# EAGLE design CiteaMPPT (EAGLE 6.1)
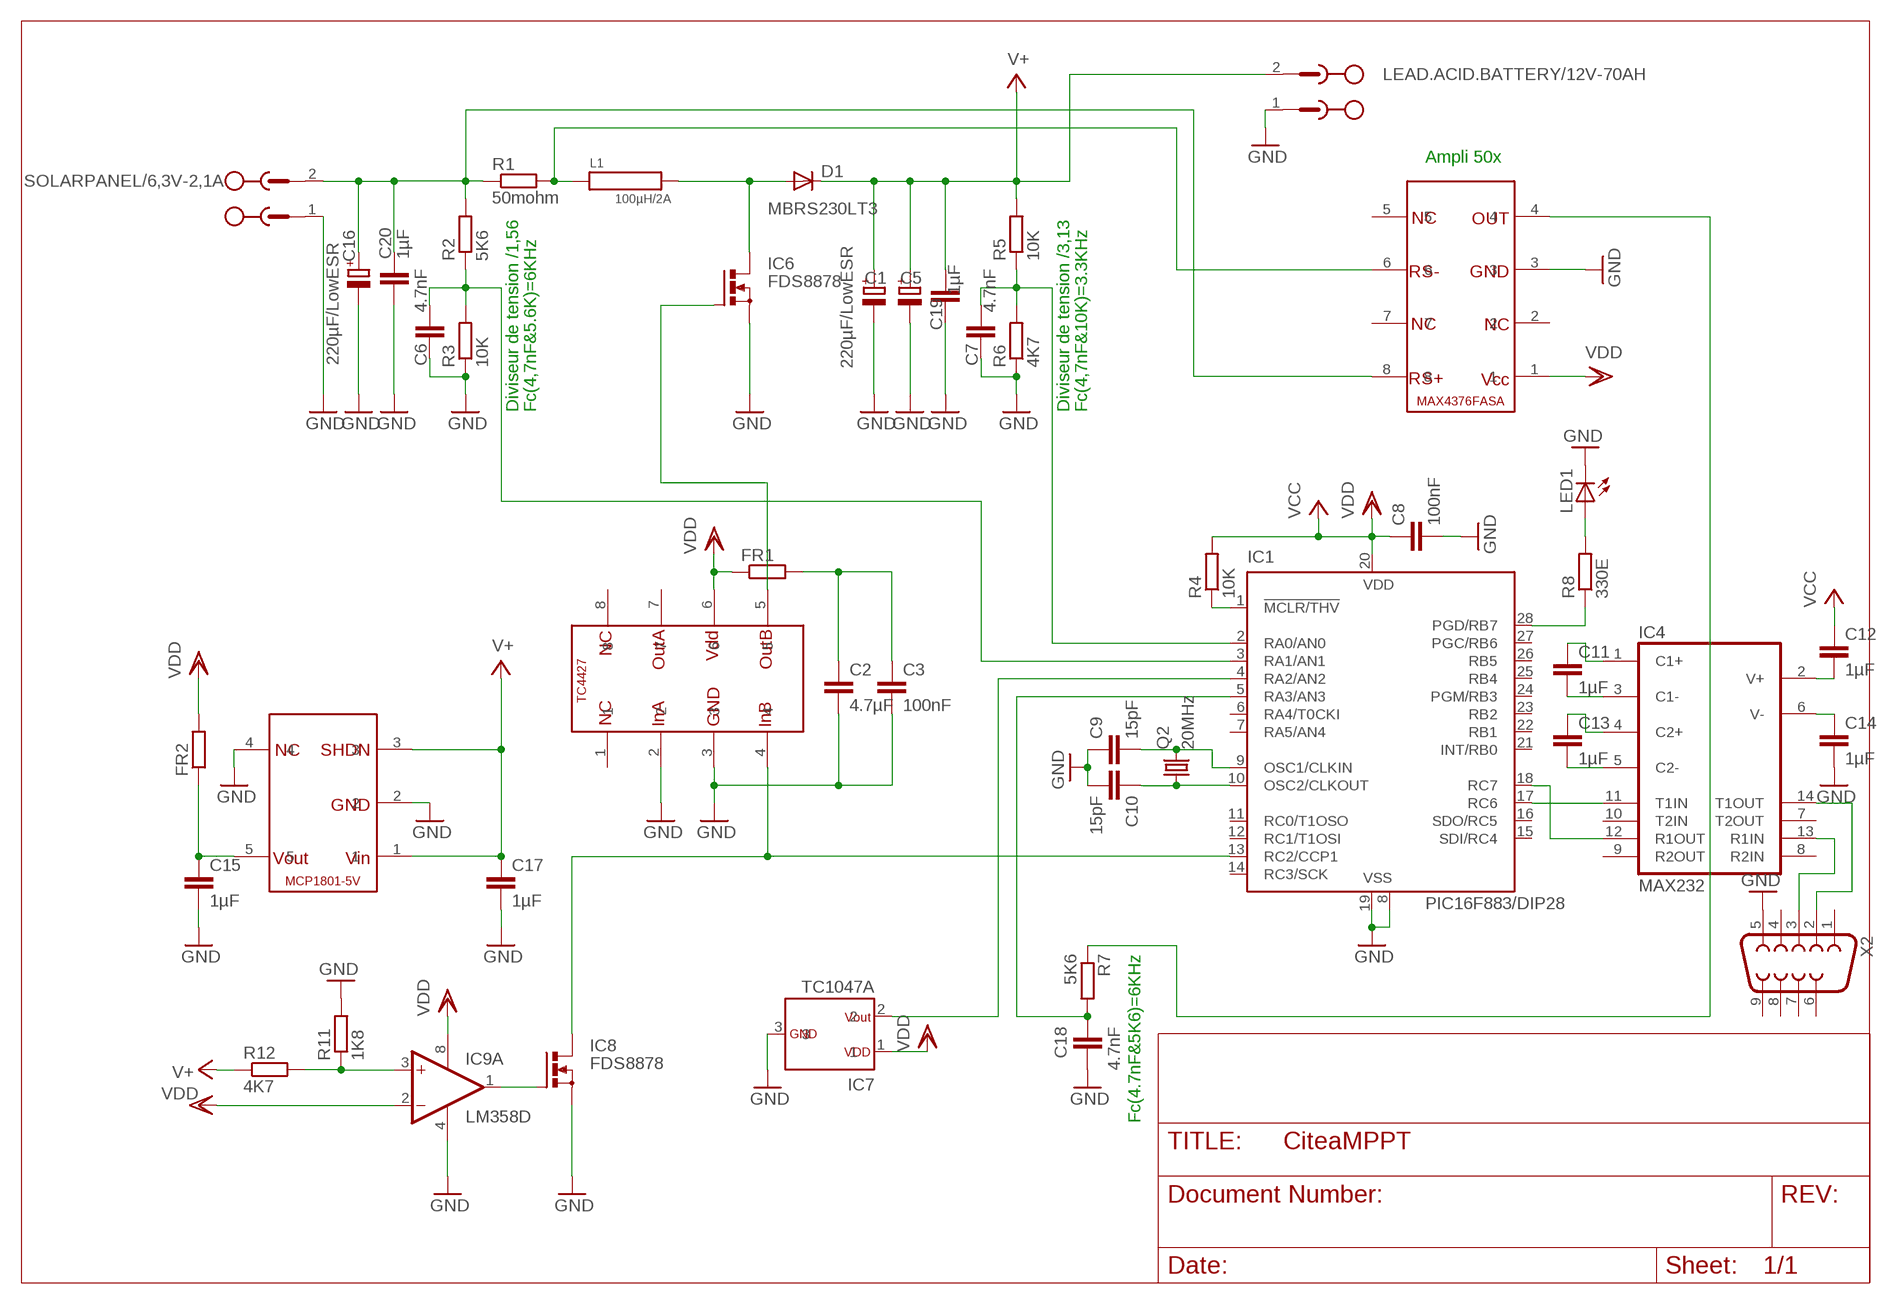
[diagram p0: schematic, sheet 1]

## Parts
C1  220µF/LowESR  CPOL-EUE3.5-8  [E3,5-8]
C2  4.7µF  C-EUC0805  [C0805]
C3  100nF  C-EUC0805  [C0805]
C5  220µF/LowESR  CPOL-EUE3.5-8  [E3,5-8]
C6  4.7nF  C-EUC0805  [C0805]
C7  4.7nF  C-EUC0805  [C0805]
C8  100nF  C-EUC0805  [C0805]
C9  15pF  C-EUC0805  [C0805]
C10  15pF  C-EUC0805  [C0805]
C11  1µF  C-EUC0805  [C0805]
C12  1µF  C-EUC0805  [C0805]
C13  1µF  C-EUC0805  [C0805]
C14  1µF  C-EUC0805  [C0805]
C15  1µF  C-EUC0805  [C0805]
C16  220µF/LowESR  CPOL-EUE3.5-8  [E3,5-8]
C17  1µF  C-EUC0805  [C0805]
C18  4.7nF  C-EUC0805  [C0805]
C19  1µF  C-EUC0805  [C0805]
C20  1µF  C-EUC0805  [C0805]
D1  MBRS230LT3  DIODE-SMB  [SMB]
FR1  R-EU_M0805  [M0805]
FR2  R-EU_M0805  [M0805]
IC1  PIC16F883/DIP28  PIC16F872P  [DIL28-3]
IC2  MAX4376  [MAX4376]
IC3  TC4427  [TC4427]
IC4  MAX232  [DIL16]
IC5  MCP1801-5V  [MCP1801-5V]
IC6  FDS8878  [FDS8878]
IC7  TC1047A  [TC1047A]
IC8  FDS8878  [FDS8878]
IC9  LM358D  [SO08]
L1  100µH/2A  WE/INDUCTOR/SMD/.100  [WE.100]
LEAD.ACID.BATTERY/12V-70AH  CONPHENIX  [CONPHENIX]
LED1  LEDCHIPLED_1206  [CHIPLED_1206]
Q2  20MHz  CRYSTALHC49S  [HC49/S]
R1  50mohm  R-EU_R1206  [R1206]
R2  5K6  R-EU_M0805  [M0805]
R3  10K  R-EU_M0805  [M0805]
R4  10K  R-EU_M0805  [M0805]
R5  10K  R-EU_M0805  [M0805]
R6  4K7  R-EU_M0805  [M0805]
R7  5K6  R-EU_M0805  [M0805]
R8  330E  R-EU_M0805  [M0805]
R11  1K8  R-EU_M0805  [M0805]
R12  4K7  R-EU_M0805  [M0805]
SOLARPANEL/6,3V-2,1A  CONPHENIX  [CONPHENIX]
X2  F09VP  [F09VP]

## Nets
GND: C1.- C2.2 C3.2 C5.- C6.2 C7.2 C8.2 C9.1 C10.2 C14.2 C15.2 C16.- C17.2 C18.1 C19.2 C20.2 IC1.8(VSS) IC1.19(VSS) IC2.3 IC3.2 IC3.3 IC5.2 IC5.4 IC6.1 IC6.2 IC6.3 IC7.3 IC8.1 IC8.2 IC8.3 IC9.4(P:V-) LEAD.ACID.BATTERY/12V-70AH.1 LED1.C R3.1 R6.1 R11.2 SOLARPANEL/6,3V-2,1A.1 X2.5
N$1: C6.1 IC1.3(RA1/AN1) R2.1 R3.2
N$2: IC2.6 L1.2 R1.2
N$3: C16.+ C20.1 IC2.8 R1.1 R2.2 SOLARPANEL/6,3V-2,1A.2
N$4: D1.A IC6.5 IC6.6 IC6.7 IC6.8 L1.1
N$5: IC8.4 IC9.1(A:OUT)
N$6: LED1.A R8.2
N$7: C9.2 IC1.9(OSC1/CLKIN) Q2.2
N$8: C18.2 IC1.5(RA3/AN3) R7.2
N$9: C7.1 IC1.2(RA0/AN0) R5.1 R6.2
N$10: IC1.13(RC2/CCP1) IC3.4 IC8.5 IC8.6 IC8.7 IC8.8
N$11: IC1.4(RA2/AN2) IC7.2
N$12: IC1.28(PGD/RB7) R8.1
N$13: IC2.4 R7.1
N$14: C10.1 IC1.10(OSC2/CLKOUT) Q2.1
N$15: C11.2 IC4.3(C1-)
N$16: C11.1 IC4.1(C1+)
N$17: C13.1 IC4.4(C2+)
N$18: C13.2 IC4.5(C2-)
N$19: C12.2 IC4.2(V+)
N$20: C14.1 IC4.6(V-)
N$21: IC1.18(RC7) IC4.12(R1OUT)
N$22: IC1.17(RC6) IC4.11(T1IN)
N$23: IC4.13(R1IN) X2.3
N$24: IC4.14(T1OUT) X2.2
N$25: C2.1 C3.1 FR1.2
N$26: IC3.5 IC6.4
N$27: IC1.1(!MCLR/THV) R4.1
N$28: C15.1 FR2.1 IC5.5
N$29: IC9.3(A:+IN) R11.1 R12.2
V+: C1.+ C5.+ C17.1 C19.1 D1.C IC5.1 IC5.3 LEAD.ACID.BATTERY/12V-70AH.2 R5.2 R12.1
VCC: C8.1 C12.1 IC1.20(VDD) R4.2 ; supply symbol labelled VDD
VDD: FR1.1 FR2.2 IC2.1 IC3.6 IC7.1 IC9.2(A:-IN) IC9.8(P:V+)
Unconnected: IC1.6(RA4/T0CKI) IC1.7(RA5/AN4) IC1.11(RC0/T1OSO) IC1.12(RC1/T1OSI) IC1.14(RC3/SCK) IC1.15(SDI/RC4) IC1.16(SDO/RC5) IC1.21(INT/RB0) IC1.22(RB1) IC1.23(RB2) IC1.24(PGM/RB3) IC1.25(RB4) IC1.26(RB5) IC1.27(PGC/RB6) IC2.2 IC2.5 IC2.7 IC3.1 IC3.7 IC3.8 IC4.7(T2OUT) IC4.8(R2IN) IC4.9(R2OUT) IC4.10(T2IN) IC9.5(B:+IN) IC9.6(B:-IN) IC9.7(B:OUT) X2.1 X2.4 X2.6 X2.7 X2.8 X2.9

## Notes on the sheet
- Ampli 50x
- Diviseur de tension /1,56 | Fc(4,7nF&5.6K)=6KHz | Diviseur de tension /3,13 | Fc(4,7nF&10K)=3.3KHz
- Fc(4.7nF&5K6)=6KHz

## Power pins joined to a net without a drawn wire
GND: IC4.15(GND)
VCC: IC4.16(VCC)

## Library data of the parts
C1 C5 C16 = rcl:CPOL-EU: POLARIZED CAPACITOR, European symbol
C2 C3 C6-C15 C17-C20 = rcl:C-EU: CAPACITOR, European symbol
D1 = diode:DIODE-: DIODE
FR1 FR2 R1-R8 R11 R12 = rcl:R-EU_: RESISTOR, European symbol
IC1 = microchip:PIC16*872: MICROCONTROLLER flash type; MF: MICROCHIP; MPN: PIC16F872-I/SP; OC_FARNELL: 9761012; OC_NEWARK: 12C1945
IC2 = solarRegulator:MAX4376
IC3 = solarRegulator:TC4427
IC4 = maxim:MAX232: RS232 TRANSEIVER; MF: MAXIM; MPN: MAX232ACPE+; OC_FARNELL: 9723773; OC_NEWARK: 68K4544
IC5 = solarRegulator:MCP1801-5V
IC6 IC8 = solarRegulator:FDS8878
IC7 = solarRegulator:TC1047A
IC9 = linear:LM358: OP AMP also LM158; LM258; LM2904 Source: http://cache.national.com/ds/LM/LM158.pdf
L1 = solarRegulator:WE/INDUCTOR/SMD/.100
LEAD.ACID.BATTERY/12V-70AH SOLARPANEL/6,3V-2,1A = solarRegulator:CONPHENIX
LED1 = led:LED: LED
Q2 = crystal:CRYSTAL: CRYSTAL; OC_FARNELL: 1667008; OC_NEWARK: unknown
X2 = con-subd:F09: SUB-D; OC_FARNELL: unknown; OC_NEWARK: unknown

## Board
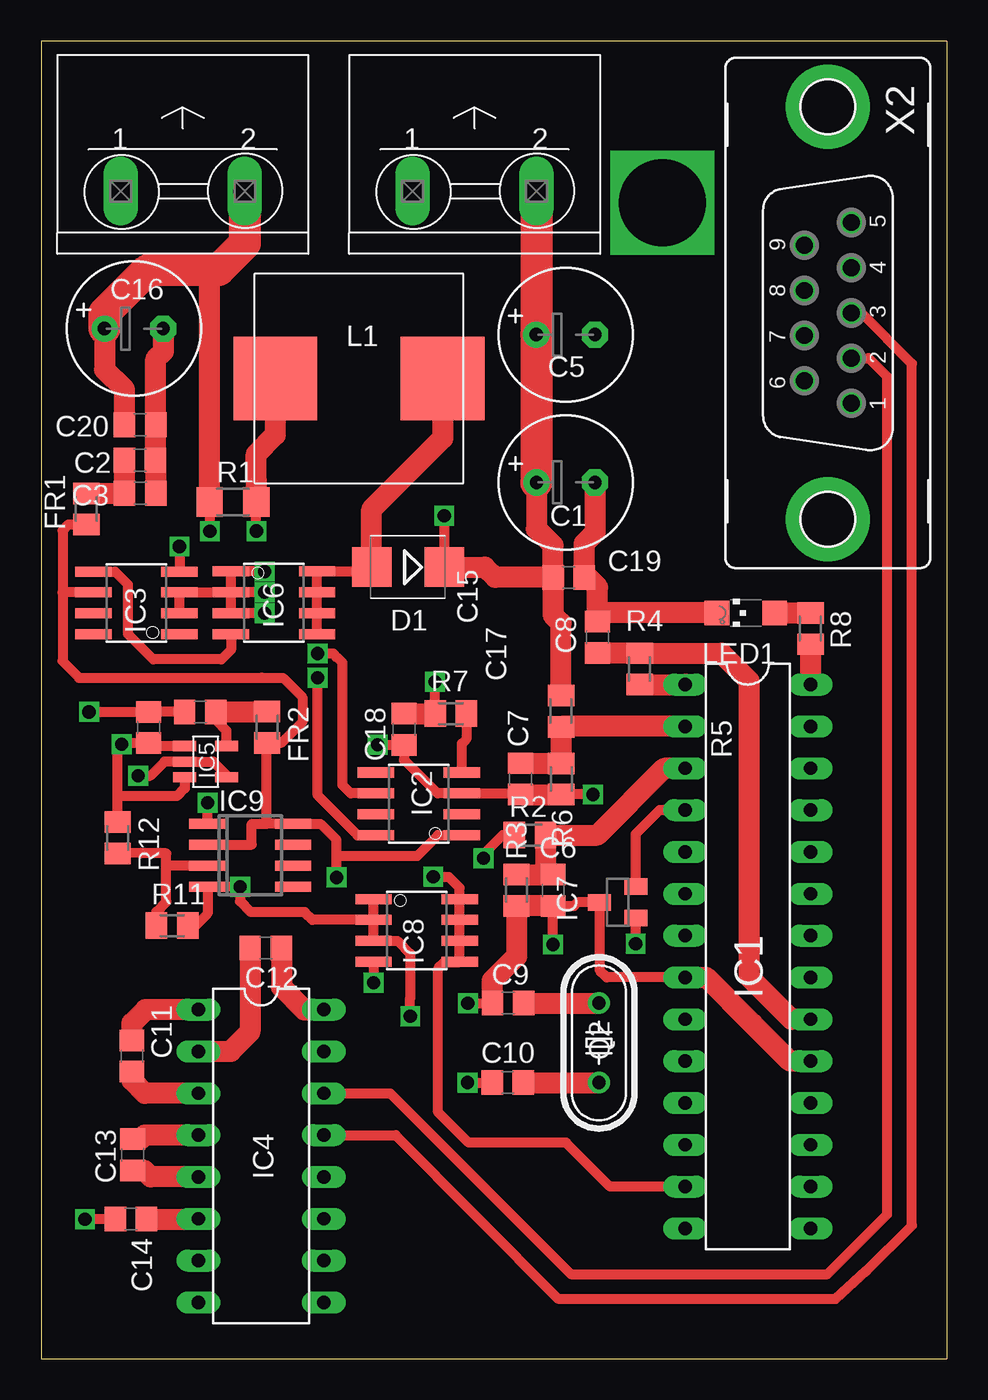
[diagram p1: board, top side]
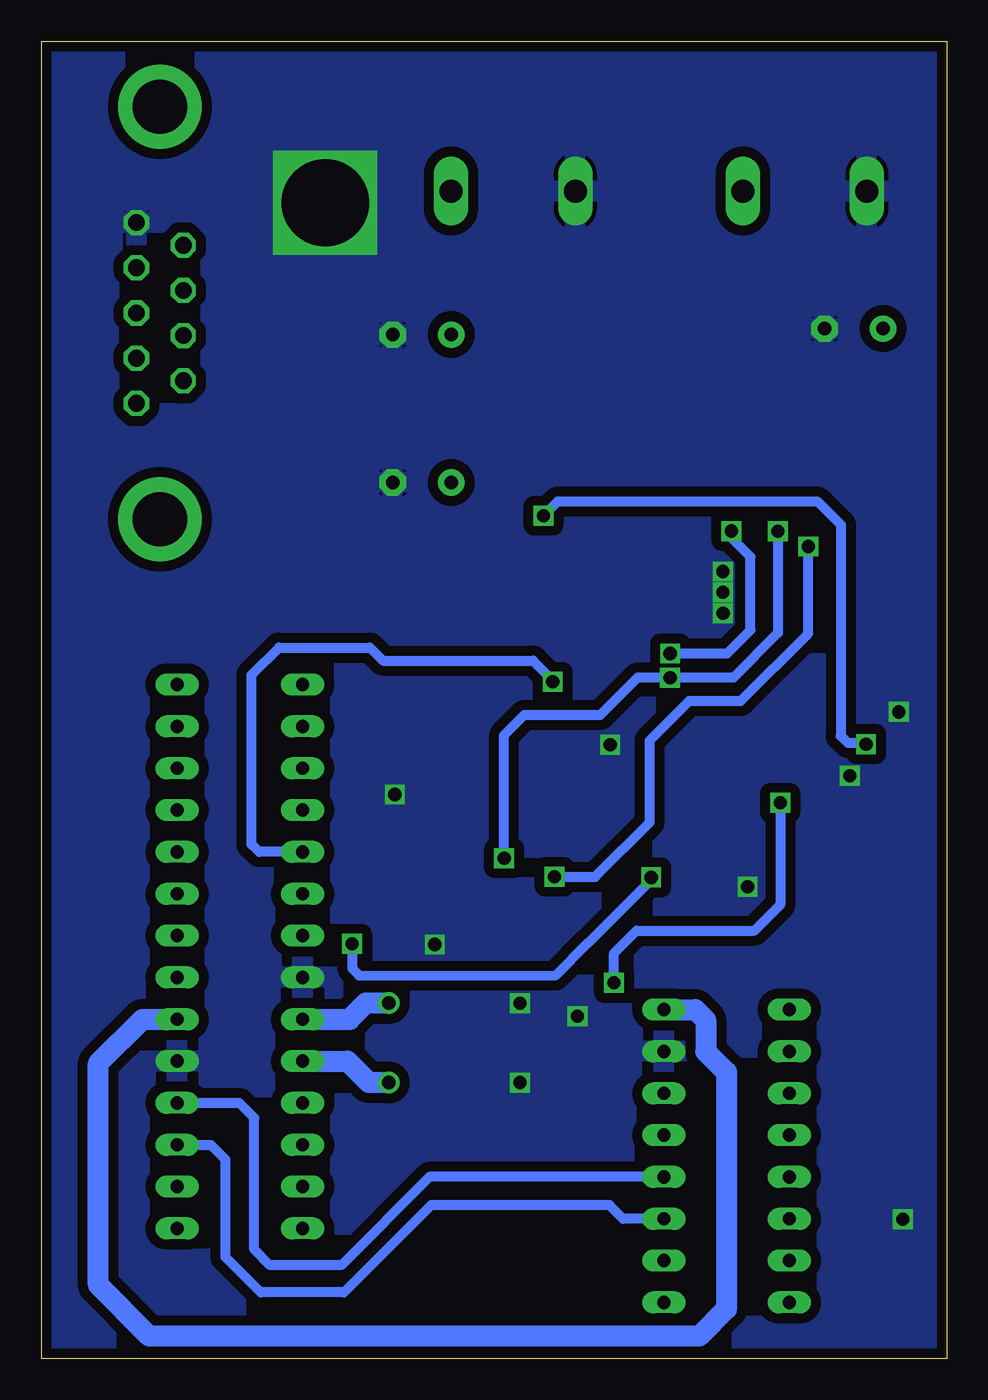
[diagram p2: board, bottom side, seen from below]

Size 55 x 80 mm. Coordinates in mm from the lower left corner, seen from the top.
Outline: 0,0 55,0 55,80 0,80 0,0
Copper layers (1*16): Top 0.035mm / dielectric 1.5mm / Bottom 0.035mm
Design rules: minimum track width 10mil, minimum drill 24mil, track to track 8mil, track to pad 8mil, pad to pad 8mil, via to via 8mil, smd to smd 8mil, copper to edge 10mil, drill to drill 8mil, minimum pad ring 10mil, minimum via ring 8mil, stop-mask expansion 4mil, vias tented up to drill 0mil, thermal gap 10mil

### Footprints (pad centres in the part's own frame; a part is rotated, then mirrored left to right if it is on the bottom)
E3,5-8 = drill 0.813 pad 1.6: + -1.778,0 | drill 0.813 pad 1.6 octagon: - 1.778,0
C0805 = smd 1.3 x 1.5: 1 -0.95,0; 2 0.95,0
SMB = smd 2.4 x 2.4: A 2.2,0; C -2.2,0
M0805 = smd 1.3 x 1.6: 1 -0.95,0; 2 0.95,0
DIL28-3 = drill 0.813 long: 1 -16.51,-3.81; 2 -13.97,-3.81; 3 -11.43,-3.81; 4 -8.89,-3.81; 5 -6.35,-3.81; 6 -3.81,-3.81; 7 -1.27,-3.81; 8 1.27,-3.81; 9 3.81,-3.81; 10 6.35,-3.81; 11 8.89,-3.81; 12 11.43,-3.81; 13 13.97,-3.81; 14 16.51,-3.81; 15 16.51,3.81; 16 13.97,3.81; 17 11.43,3.81; 18 8.89,3.81; 19 6.35,3.81; 20 3.81,3.81; 21 1.27,3.81; 22 -1.27,3.81; 23 -3.81,3.81; 24 -6.35,3.81; 25 -8.89,3.81; 26 -11.43,3.81; 27 -13.97,3.81; 28 -16.51,3.81
MAX4376 = smd 2.21 x 0.61: 1 -2.616,1.905; 2 -2.616,0.635; 3 -2.616,-0.635; 4 -2.616,-1.905; 5 2.616,-1.905; 6 2.616,-0.635; 7 2.616,0.635; 8 2.616,1.905
TC4427 = smd 2.21 x 0.61: 1 -2.616,1.905; 2 -2.616,0.635; 3 -2.616,-0.635; 4 -2.616,-1.905; 5 2.616,-1.905; 6 2.616,-0.635; 7 2.616,0.635; 8 2.616,1.905
DIL16 = drill 0.813 long: 1 -8.89,-3.81; 2 -6.35,-3.81; 3 -3.81,-3.81; 4 -1.27,-3.81; 5 1.27,-3.81; 6 3.81,-3.81; 7 6.35,-3.81; 8 8.89,-3.81; 9 8.89,3.81; 10 6.35,3.81; 11 3.81,3.81; 12 1.27,3.81; 13 -1.27,3.81; 14 -3.81,3.81; 15 -6.35,3.81; 16 -8.89,3.81
MCP1801-5V = smd 0.61 x 1.397: 1 -0.953,-1.27; 2 0,-1.27; 3 0.953,-1.27; 4 0.953,1.27; 5 -0.953,1.27
FDS8878 = smd 2.21 x 0.61: 1 -2.616,1.905; 2 -2.616,0.635; 3 -2.616,-0.635; 4 -2.616,-1.905; 5 2.616,-1.905; 6 2.616,-0.635; 7 2.616,0.635; 8 2.616,1.905
TC1047A = smd 1 x 1.4: 1 -0.95,-1.1; 2 0.95,-1.1; 3 0,1.1
SO08 = smd 0.6 x 2.2: 1 -1.905,-2.6; 2 -0.635,-2.6; 3 0.635,-2.6; 4 1.905,-2.6; 5 1.905,2.6; 6 0.635,2.6; 7 -0.635,2.6; 8 -1.905,2.6
WE.100 = smd 5.08 x 5.08: 1 -5.08,0; 2 5.08,0
CONPHENIX = drill 1.397 long: 1 4.405,0; 2 -3.135,0
CHIPLED_1206 = smd 1.5 x 1.5: A 0,-1.75; C 0,1.75
HC49/S = drill 0.813: 1 -2.413,0; 2 2.413,0
R1206 = smd 1.6 x 1.803: 1 -1.422,0; 2 1.422,0
F09VP = drill 1.016 octagon: 1 5.486,1.422; 2 2.743,1.422; 3 0,1.422; 4 -2.743,1.422; 5 -5.486,1.422; 6 4.115,-1.422; 7 1.372,-1.422; 8 -1.372,-1.422; 9 -4.115,-1.422 | drill 3.302 pad 5.08: G1 -12.522,0; G2 12.522,0

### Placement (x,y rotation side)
C1  31.87,53.21 0 top
C2  6,54.56 0 top
C3  6.02,52.55 0 top
C5  31.86,62.18 0 top
C6  31.11,28.45 270 top
C7  29.11,35.21 270 top
C8  33.79,43.81 90 top
C9  28.36,21.6 0 top
C10  28.34,16.77 180 top
C11  5.52,18.38 270 top
C12  13.64,24.94 180 top
C13  5.56,12.39 270 top
C14  5.46,8.48 180 top
C15  9.67,39.28 180 top
C16  5.63,62.54 0 top
C17  6.54,38.33 90 top
C18  22.04,38.22 90 top
C19  32.05,47.44 0 top
C20  6.01,56.71 0 top
D1  22.27,48.07 180 top
FR1  2.75,51.6 90 top
FR2  13.73,38.34 270 top
IC1  42.93,24.43 270 top
IC2  22.94,33.69 180 top
IC3  5.78,45.89 180 top
IC4  13.36,12.31 270 top
IC5  9.99,36.25 270 top
IC6  14.14,45.9 0 top
IC7  35.02,27.72 90 top
IC8  22.81,26.01 0 top
IC9  12.7,30.58 270 top
L1  19.31,59.52 180 top
LEAD.ACID.BATTERY/12V-70AH  26.96,70.9 180 top
LED1  42.8,45.29 90 top
Q2  33.88,19.19 90 top
R1  11.65,52.02 0 top
R2  29.68,31.8 180 top
R3  28.87,28.45 90 top
R4  36.35,41.89 90 top
R5  31.59,39.32 90 top
R6  31.59,35.2 90 top
R7  24.88,39.17 180 top
R8  46.73,44.33 90 top
R11  7.96,26.3 0 top
R12  4.65,31.63 270 top
SOLARPANEL/6,3V-2,1A  9.24,70.9 180 top
X2  47.79,63.5 270 top

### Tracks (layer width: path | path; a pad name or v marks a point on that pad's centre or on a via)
GND  (via drill 0.8, 5.3)
  Top 0.61: IC6.2 IC6.3 11.56,45.26 11.56,45.27 | IC6.2 IC6.1 | IC3.2 IC3.3 IC6.2 | v13.58,46.53 12.42,46.54 12.43,46.53 | 12.43,46.54 12.43,46.53 | IC6.2 12.43,46.53 | v13.58,47.8 IC6.1 | IC6.1 | v13.58,45.27 11.56,45.27 | 11.56,45.27 11.56,45.31 | IC5.4 11.26,35.44 10.45,36.26 IC5.2 7.5,36.26 6.65,35.41 v5.89,35.41 | R11.2 9.37,26.3 10.1,27.03 IC9.4 | C15.2 8.7,39.29 C17.2 | C7.2 29.06,34.31 29.06,34.34 29.05,34.33 IC2.3 24.08,34.33 22.04,36.37 C18.1 v20.43,37.27 | IC9.4 v12.08,28.67 12.08,27.77 12.74,27.12 16.01,27.12 16.48,26.65 IC8.2 | 10.09,28.67 IC9.4 | IC9.4 | 6.53,39.28 | 6.53,39.28 C17.2 | C17.2 | v25.92,21.59 27.39,21.59 27.41,21.59 C9.1 | v25.91,16.77 C10.2 | IC8.2 IC8.3 21.65,25.38 22.42,24.6 22.42,21.9 | IC8.2 20.2,27.79 20.17,27.79 20.17,27.74 | IC8.2 IC8.1 20.19,27.9 20.2,27.9 | IC1.8 34.36,23.16 33.92,23.6 33.92,23.61 IC7.3 32.59,27.72 32.37,27.5 C6.2 31.09,27.48 v31.09,25.15 | v33.52,34.26 31.58,34.26 31.55,34.3 R6.1 | 22.42,21.9 22.41,21.9 | v22.42,20.81 22.42,21.9 22.42,21.91 22.42,21.9 | v2.91,39.28 C17.2 | C17.2 | C14.2 v2.67,8.48 v2.66,8.48
  Top 1.27: C1.- 33.64,50.16 33,49.51 C19.2 33.2,47.44 33.81,46.84 33.79,46.82 C8.2 33.76,44.78 33.76,44.87 34.18,45.29 LED1.C | C16.- 7.41,61.16 6.96,60.7 C20.2 C2.2 6.95,52.56 C3.2 | C15.2 | C7.2 R6.1 | C6.2 R3.1 28.87,24.43 27.41,22.97 C9.1 | IC1.8 40.4,23.16 43.2,20.36 | IC1.19 45.48,18.08 43.2,20.36 | 43.2,20.36 | 43.2,20.36 43.2,20.35
  other vias: 37.74,70.19
  pour Bottom (isolate 0.61): 1,79 54,79 54,1 1,1
N$1
  Top 1.27: R3.2 31.12,29.4 31.14,29.39 C6.1 30.72,29.4 30.63,29.49 R2.1 33.78,31.8 37.84,35.86 IC1.3
N$2  (via drill 0.8)
  Top 0.61: v13.07,50.26 13.07,50.33 R1.2 | IC2.6 18.81,34.33 18.3,34.84 18.3,41.97 | 18.3,41.97 | v16.79,42.82 17.74,42.82 18.02,42.55 | 18.02,42.55 18.03,42.55 | 18.3,41.97 18.3,42.27 18.02,42.55
  Top 1.27: R1.2 13.07,54.94 14.23,56.09 L1.2
  Bottom 0.61: v16.79,42.82 13.32,42.82 11.91,44.24 11.91,48.69 13.07,49.85 v13.07,50.26 13.07,50.33
N$3  (via drill 0.8)
  Top 0.61: v10.25,50.25 10.25,50.35 10.25,52.03 10.25,52.02 R1.1 | IC2.8 19.21,31.79 16.8,34.2 v16.8,41.36 | v26.88,30.39 26.88,30.64 28.03,31.8 R2.2
  Top 1.27: R1.1 10.23,65.72 10.63,66.12 | C20.1 5.06,58.86 3.86,60.06 C16.+
  Top 1.93: C16.+ 3.86,63.5 6.48,66.12 10.63,66.12 10.79,66.12 12.37,67.7 SOLARPANEL/6,3V-2,1A.2
  Bottom 0.61: v10.25,50.25 10.24,44.07 12.95,41.36 16.64,41.36 v16.8,41.36 18.77,41.36 21.03,39.1 25.64,39.1 26.88,37.87 v26.88,30.39
N$4
  Top 0.61: IC6.5 IC6.6 IC6.7 IC6.8 19.81,47.8 20,48 | 20,48 | 20,48 D1.A
  Top 1.27: D1.A 20.07,51.57 24.39,55.88 L1.1
N$5  (via drill 0.8)
  Top 0.61: IC8.4 v20.2,22.83 v20.2,22.82 | IC9.1 v10.1,33.75 v10.11,33.76
  Bottom 0.61: v20.2,22.82 20.2,24.63 18.84,25.99 11.67,25.99 10.11,27.55 v10.11,33.76
N$6
  Top 1.27: LED1.A R8.2
N$7
  Top 1.27: C9.2 Q2.2 33.9,21.61 Q2.2
  Bottom 1.27: Q2.2 35.28,21.6 36.26,20.62 IC1.9
N$8  (via drill 0.8)
  Top 0.61: C18.2 | R7.2 v23.93,41.1
  Top 1.27: C18.2 R7.2
  Bottom 0.61: IC1.5 41.76,30.78 42.22,31.24 42.22,41.52 40.56,43.18 35.02,43.18 34.23,42.39 25.12,42.39 23.93,41.2 v23.93,41.1
N$9
  Top 1.27: C7.1 31.54,36.16 31.55,36.17 31.58,36.17 R6.2 R5.1 31.61,38.4 IC1.2
N$10  (via drill 0.8)
  Top 0.61: IC8.8 IC8.7 IC8.6 IC8.5 25.41,24.09 24.49,24.09 24.11,23.71 24.11,14.96 25.96,13.12 31.89,13.12 34.55,10.46 IC1.13 | IC8.8 | IC8.8 | IC8.8 | v8.4,49.32 IC3.4 | IC3.4 | IC3.4 | v23.82,29.27 24.75,29.27 25.43,28.59 IC8.8
  Bottom 0.61: v8.4,49.32 8.4,49.3 8.4,44.03 12.52,39.93 15.64,39.93 18.03,37.54 18.03,32.59 21.35,29.27 v23.82,29.27
N$11
  Top 0.61: IC1.4 37.56,33.32 36.12,31.88 IC7.2
N$12
  Top 1.27: R8.1 46.73,40.95 IC1.28
N$13
  Top 0.61: IC2.4 25.56,37.35 25.83,37.63 R7.1
N$14
  Top 1.27: C10.1 Q2.1 | Q2.1
  Bottom 1.27: Q2.1 35.09,16.77 36.39,18.08 IC1.10
N$15
  Top 1.27: C11.2 5.52,16.9 6.3,16.12 IC4.3
N$16
  Top 1.27: C11.1 5.52,20.39 6.34,21.2 IC4.1
N$17
  Top 1.27: C13.1 6.05,13.34 6.29,13.58 IC4.4
N$18
  Top 1.27: C13.2 6.27,11.44 6.66,11.04 IC4.5
N$19
  Top 1.27: C12.2 12.69,19.84 11.51,18.66 IC4.2
N$20
  Top 1.27: C14.1 9.55,8.48 9.57,8.5 IC4.6
N$21
  Bottom 0.61: IC4.12 31.41,11.04 36.76,5.69 41.11,5.69 42.06,6.64 42.06,14.63 42.97,15.54 IC1.18
N$22
  Bottom 0.61: IC4.11 19.65,8.5 20.48,9.33 31.31,9.33 36.61,4.03 41.66,4.03 43.8,6.17 43.8,12.1 44.7,13 IC1.17
N$23
  Top 0.61: IC4.13 21.54,13.58 31.39,3.65 48.26,3.64 50.14,5.34 52.89,8.09 52.89,60.42 49.82,63.5 X2.3
N$24
  Top 0.61: IC4.14 21.2,16.12 32.18,5.14 47.77,5.14 51.39,8.77 51.39,59.63 50.27,60.76 X2.2
N$25
  Top 1.27: FR1.2 C3.1 5.07,54.54 C2.1
N$26
  Top 0.61: IC6.4 11.53,43.04 10.95,42.46 6.82,42.46 5.28,44 5.28,47.01 4.49,47.8 IC3.5
N$27
  Top 1.27: R4.1 IC1.1 39.14,40.96 | 39.14,40.96 | 39.14,40.96 IC1.1
N$28
  Top 0.61: C15.1 10.62,38.79 11.26,38.15 IC5.5
  Top 1.27: C15.1 13.71,39.28 FR2.1
N$29
  Top 0.61: R11.1 7.01,27.15 7.61,27.75 7.61,29.94 | 7.61,29.94 7.61,30.69 6.04,30.69 6.04,30.72 R12.2 | IC9.3 7.61,29.94
V+  (via drill 0.8)
  Top 0.61: IC5.1 6.71,37.21 C17.1 6.55,37.39 4.96,37.39 v4.89,37.32 4.64,37.08 4.64,34.04 | R12.1 4.64,34.04 | IC5.3 8.72,34.63 8.26,34.17 4.77,34.17 4.64,34.04 | v24.48,51.18 24.48,48.12 24.47,48.1 D1.C
  Top 1.27: C1.+ 30.09,50.39 31.1,49.38 C19.1 | D1.C 26.96,48.07 27.59,47.44 C19.1 | R5.2 31.59,44.67 31.1,45.16 C19.1
  Top 1.93: LEAD.ACID.BATTERY/12V-70AH.2 30.1,62.47 C5.+ C1.+
  Bottom 0.61: v24.48,51.18 23.61,52.06 7.85,52.06 6.42,50.63 6.43,50.63 6.43,37.83 5.99,37.39 4.96,37.39 v4.89,37.32
VCC
  Top 1.27: C8.1 36.33,42.86 R4.2 41.33,42.84 43,41.16 43,23.19 45.58,20.62 IC1.20 | C12.1 14.59,22.58 15.98,21.19 17.16,21.19 IC4.16
  Bottom 1.27: IC4.16 15.26,21.2 14.63,20.57 14.63,18.66 13.38,17.41 13.38,3.03 15.02,1.38 48.42,1.38 51.52,4.48 51.52,17.93 48.84,20.62 IC1.20
VDD  (via drill 0.8)
  Top 0.61: 13.69,32.48 IC9.8 16.97,32.48 17.94,31.51 17.94,30.54 | 13.69,32.48 13.7,37.4 13.69,37.41 13.71,37.41 | 13.71,37.41 FR2.2 | IC2.1 25.55,31.8 24.1,31.8 22.85,30.54 17.94,30.54 | 13.71,37.41 14.61,37.41 15.88,38.68 15.88,40.16 14.69,41.35 13.41,41.35 | FR1.1 1.65,50.65 1.3,50.29 1.3,46.53 | 1.3,46.53 1.3,42.35 2.3,41.35 13.41,41.35 | 13.41,41.35 13.42,41.35 | IC3.6 1.3,46.53 | IC9.2 12.79,31.21 12.79,32.47 13.69,32.48 | v17.94,29.23 17.94,30.54 | IC7.1 v36.11,25.2
  Bottom 0.61: v17.94,29.23 17.94,29.09 21.83,25.2 21.85,25.19 23.76,23.27 35.69,23.29 36.11,23.71 v36.11,25.2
